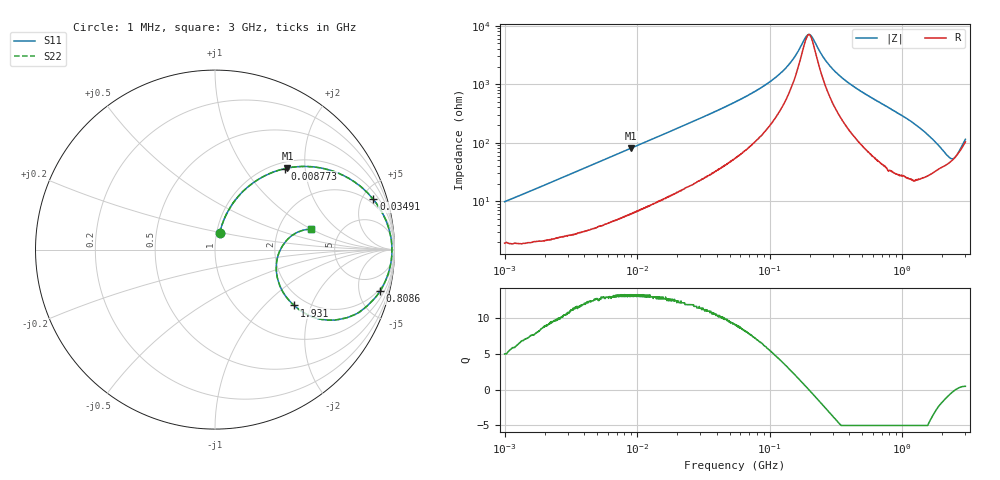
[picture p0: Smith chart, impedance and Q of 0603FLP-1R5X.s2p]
!s-Parameter Generated by FASTRON Sdn. Bhd.
!FASTRON P/N : 0603FLP-1R5X
!Keysight Technologies: E4991B_MY54100416_A.01.15
!Date: Tue Dec 02 13:00:19 2025
!Version  :Rev00  Tue Dec 02 13:00:19 2025
!Data & Calibration Information:
!Freq  S11  S21  S12  S22
!PortZ  Port1:50+j0  Port2:50+j0
!When reading reference impedance value at option line is always used.
! Remarks : This data is being provided solely for informational purposes.
# Hz S dB R 50
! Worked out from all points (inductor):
!   1601 points, 1 MHz to 3 GHz, reference 50 ohm
!   read as one part in series: L = 1.52 uH near 1.041 MHz
!   highest Q = 13.3 at 9.041 MHz (marker M1), where L = 1.42 uH
!   self-resonance near 197.7 MHz
!   S11 on the Smith chart (normalised r, x): 1 MHz: 1.04, +0.19; 8.773 MHz: 1.12, +1.57; 34.91 MHz: 1.55, +6.07; 808.6 MHz: 1.68, -7.67; 1.931 GHz: 1.73, -1.52; 3 GHz: 3.06, +0.98
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1000000  -20.40 73.3  -0.20 -5.4  -0.20 -5.4  -20.40 73.3
3804036  -9.83 66.4  -0.73 -18.7  -0.73 -18.7  -9.83 66.4
8773424  -4.49 49.2  -2.40 -36.5  -2.40 -36.5  -4.49 49.2
9040831  -4.33 48.4  -2.50 -37.3  -2.50 -37.3  -4.33 48.4
1.447069e7  -2.39 36.4  -4.52 -49.2  -4.52 -49.2  -2.39 36.4
3.491183e7  -0.67 17.6  -10.40 -67.2  -10.40 -67.2  -0.67 17.6
5.504702e7  -0.35 11.1  -14.30 -72.6  -14.30 -72.6  -0.35 11.1
1.137229e8  -0.16 4.0  -22.90 -73.6  -22.90 -73.6  -0.16 4.0
1.482612e8  -0.13 2.0  -28.30 -65.8  -28.30 -65.8  -0.13 2.0
1.904091e8  -0.12 0.3  -36.60 -17.9  -36.60 -17.9  -0.12 0.3
2.083556e8  -0.12 -0.4  -36.30 24.4  -36.30 24.4  -0.12 -0.4
2.596726e8  -0.13 -1.9  -28.70 65.6  -28.70 65.6  -0.13 -1.9
3.204059e8  -0.14 -3.5  -24.00 73.4  -24.00 73.4  -0.14 -3.5
4.639993e8  -0.20 -6.8  -18.40 75.7  -18.40 75.7  -0.20 -6.8
7.925923e8  -0.44 -13.9  -12.40 71.3  -12.40 71.3  -0.44 -13.9
8.086166e8  -0.47 -14.2  -12.20 70.8  -12.20 70.8  -0.47 -14.2
1.243477e9  -1.26 -24.4  -7.61 59.4  -7.61 59.4  -1.26 -24.4
1.596974e9  -2.81 -32.7  -5.15 45.0  -5.15 45.0  -2.81 -32.7
1.931433e9  -5.35 -35.2  -3.88 29.2  -3.88 29.2  -5.35 -35.2
2.407135e9  -9.12 -10.7  -3.62 5.7  -3.62 5.7  -9.12 -10.7
2.714296e9  -7.30 10.1  -4.73 -7.5  -4.73 -7.5  -7.30 10.1
3e9  -5.25 11.9  -6.40 -13.6  -6.40 -13.6  -5.25 11.9
